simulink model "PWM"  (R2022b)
settings: Solver=ode4  StartTime=0.0  StopTime=0.1  FixedStep=1e-6  RelTol=1e-3
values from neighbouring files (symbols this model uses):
  a_s_control = 10    [PWM.m]
  a_s_portadora = 5    [PWM.m]
  f_s_control = 100    [PWM.m]
  p_s_portadora = 1/f_s_portadora    (= 0.0166666666667)    [PWM.m]
libraries: simulink x1

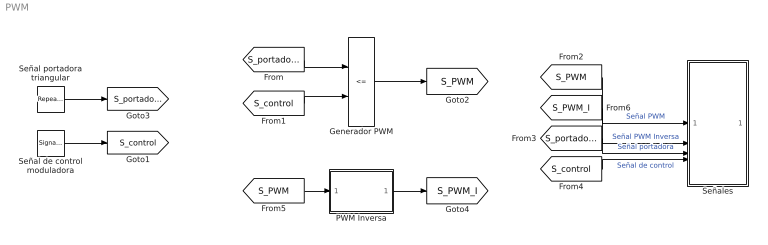
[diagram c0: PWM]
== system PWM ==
  Generador PWM : RelationalOperator  Operator=<=  OutDataTypeStr=boolean  RndMeth=Simplest
  PWM Inversa : MATLAB Function  TreatAsAtomicUnit=on
  Señal de control moduladora : SignalGenerator  Amplitude=a_s_control  Frequency=f_s_control
  Señal portadora triangular : simulink/Sources/Repeating Sequence  rep_seq_t=[0 p_s_portadora/2 p_s_portadora]  rep_seq_y=[-a_s_portadora a_s_portadora -a_s_portadora]
  Señales : Subsystem
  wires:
  Señal portadora triangular/1 -> [S_portadora]
  [S_portadora] -> Generador PWM/1
  [S_control] -> Generador PWM/2
  Señal de control moduladora/1 -> [S_control]
  Generador PWM/1 -> [S_PWM]
  [S_PWM] -> Señales/1(S_PWM)  "Señal PWM"
  [S_portadora] -> Señales/3(S_portadora)  "Señal portadora"
  [S_control] -> Señales/4(S_control)  "Señal de control"
  [S_PWM] -> PWM Inversa/1(u)
  PWM Inversa/1(y) -> [S_PWM_I]
  [S_PWM_I] -> Señales/2(S_PWM_I)  "Señal PWM Inversa"

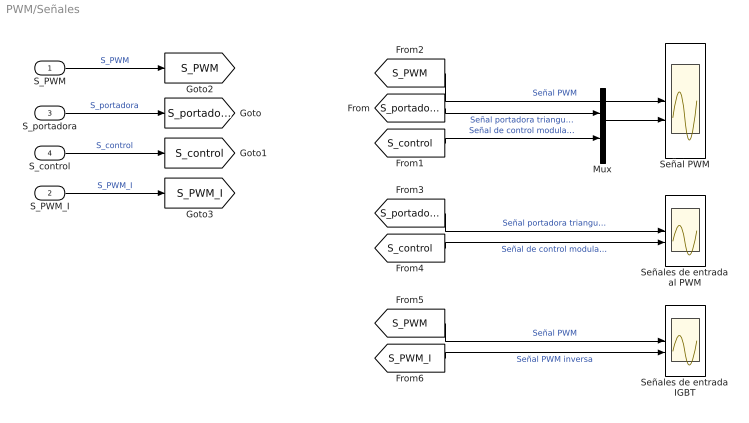
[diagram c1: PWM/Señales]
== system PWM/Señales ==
  S_PWM : Inport
  S_PWM_I : Inport  Port=2
  S_portadora : Inport  Port=3
  S_control : Inport  Port=4
  Mux : Mux  Inputs=2
  Señal PWM : Scope  NumInputPorts=2
  Señales de entrada IGBT : Scope  NumInputPorts=2
  Señales de entrada al PWM : Scope  NumInputPorts=2
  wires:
  Mux/1 -> Señal PWM/2
  S_PWM/1 -> [S_PWM]  "S_PWM"
  S_portadora/1 -> [S_portadora]  "S_portadora"
  S_control/1 -> [S_control]  "S_control"
  [S_portadora] -> Mux/1  "Señal portadora triangular"
  [S_control] -> Mux/2  "Señal de control moduladora"
  [S_PWM] -> Señal PWM/1  "Señal PWM"
  [S_control] -> Señales de entrada al PWM/2  "Señal de control moduladora"
  [S_portadora] -> Señales de entrada al PWM/1  "Señal portadora triangular"
  S_PWM_I/1 -> [S_PWM_I]  "S_PWM_I"
  [S_PWM] -> Señales de entrada IGBT/1  "Señal PWM"
  [S_PWM_I] -> Señales de entrada IGBT/2  "Señal PWM inversa"

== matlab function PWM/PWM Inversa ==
function y = fcn(u)

    if u == 1
        y = 0;
    else
        y = 1;
    end
end
